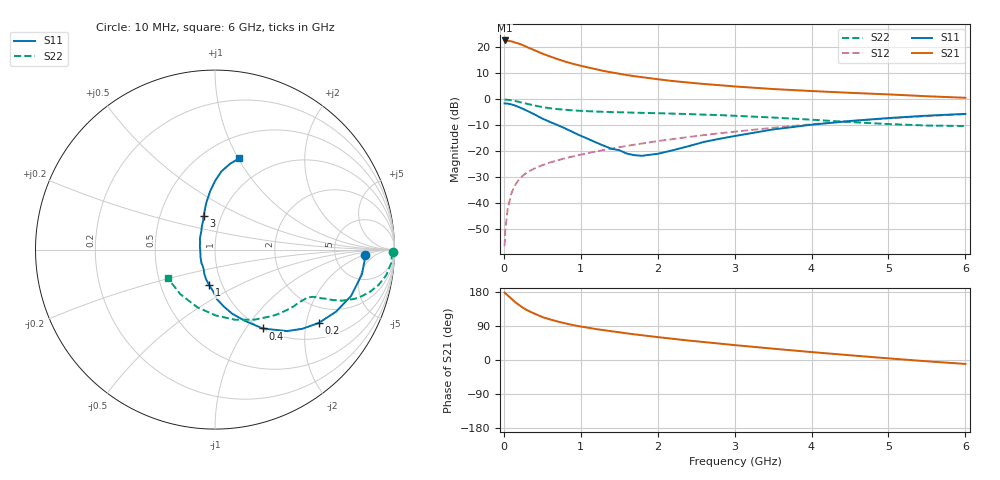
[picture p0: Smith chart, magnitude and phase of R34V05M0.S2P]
! SIEMENS Small Signal Semiconductors
! BFR181
! Si NPN RF Bipolar Junction Transistor in SOT23
! VCE = 4 V  IC = 5 mA
! Common Emitter S-Parameters:  May  1996
# GHz  S  MA  R  50
!  f  S11  S21  S12  S22
! GHz  MAG  ANG  MAG  ANG  MAG  ANG  MAG  ANG
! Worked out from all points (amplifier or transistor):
!   36 points, 10 MHz to 6 GHz, reference 50 ohm
!   highest |S21| = 22.7 dB at 10 MHz (marker M1)
!   |S21| within 3 dB of that: start of sweep to 337 MHz
!   unconditionally stable (mu >= 1): 1.144 GHz to 3.003 GHz
!   at 250 MHz: K = 0.42, MSG = 25.1 dB, |S12| = -29.3 dB
!   at 1.4 GHz: K = 1.05, MAG = 13.3 dB, |S12| = -18.9 dB
!   at 6 GHz: K = 0.86, MSG = 3.1 dB, |S12| = -5.6 dB
!   lowest NFmin = 1.55 dB at 450 MHz
!   S11 on the Smith chart (normalised r, x): 10 MHz: 11, -2; 200 MHz: 1.44, -2.37; 400 MHz: 1.00, -1.20; 1 GHz: 0.87, -0.36; 3 GHz: 0.82, +0.32; 6 GHz: 0.72, +1.01
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0.01  0.8375 -2.1  13.64 177.8  0.0015 94.9  0.9916 -0.9
0.02  0.8363 -3.8  13.37 175.9  0.0032 85.8  0.9859 -1.8
0.05  0.8302 -9.5  13.43 170.5  0.0078 84.6  0.9847 -4.4
0.1  0.8011 -18.8  13.12 161.5  0.0158 80.9  0.9639 -8.6
0.15  0.7581 -27.1  12.39 152.3  0.023 75.7  0.9314 -12.3
0.2  0.7077 -35.3  11.81 144.8  0.0292 72.9  0.8952 -15.2
0.25  0.6568 -42.2  11.04 137.7  0.0344 69.5  0.8566 -17.7
0.3  0.6063 -48.5  10.18 131.7  0.0394 68.3  0.8232 -19.5
0.4  0.5132 -58.9  8.828 122.1  0.0471 64.9  0.7629 -21.9
0.5  0.4279 -67.5  7.624 113.4  0.0542 63.8  0.7127 -23.2
0.6  0.3689 -75.1  6.712 107.1  0.0611 63.5  0.6766 -23.9
0.8  0.2756 -87.9  5.336 96.6  0.0739 62.9  0.6317 -24.9
1  0.1996 -99.5  4.445 88.3  0.0865 63.7  0.6028 -25.9
1.1  0.1725 -106.7  4.109 85.0  0.0931 64.1  0.5931 -26.5
1.3  0.1286 -119.0  3.532 78.8  0.1065 64.3  0.5772 -27.9
1.6  0.0905 -153.4  2.943 70.2  0.1276 64.2  0.5618 -30.6
2.2  0.1053 142.6  2.256 55.9  0.1728 62.6  0.5334 -37.6
3  0.1974 108.8  1.779 39.3  0.2396 58.0  0.4851 -50.0
3.5  0.2646 100.6  1.585 29.9  0.285 54.1  0.4486 -60.4
4.5  0.3843 89.8  1.34 12.5  0.3826 43.9  0.3671 -89.3
5.5  0.487 79.9  1.151 -3.4  0.4782 31.4  0.3147 -127.9
6  0.5266 75.0  1.076 -10.4  0.5219 24.4  0.3077 -149.2
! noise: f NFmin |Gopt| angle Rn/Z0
0.45  1.55  0.48  17  0.36
0.9  1.65  0.4  35  0.34
1.8  2  0.18  88  0.34
